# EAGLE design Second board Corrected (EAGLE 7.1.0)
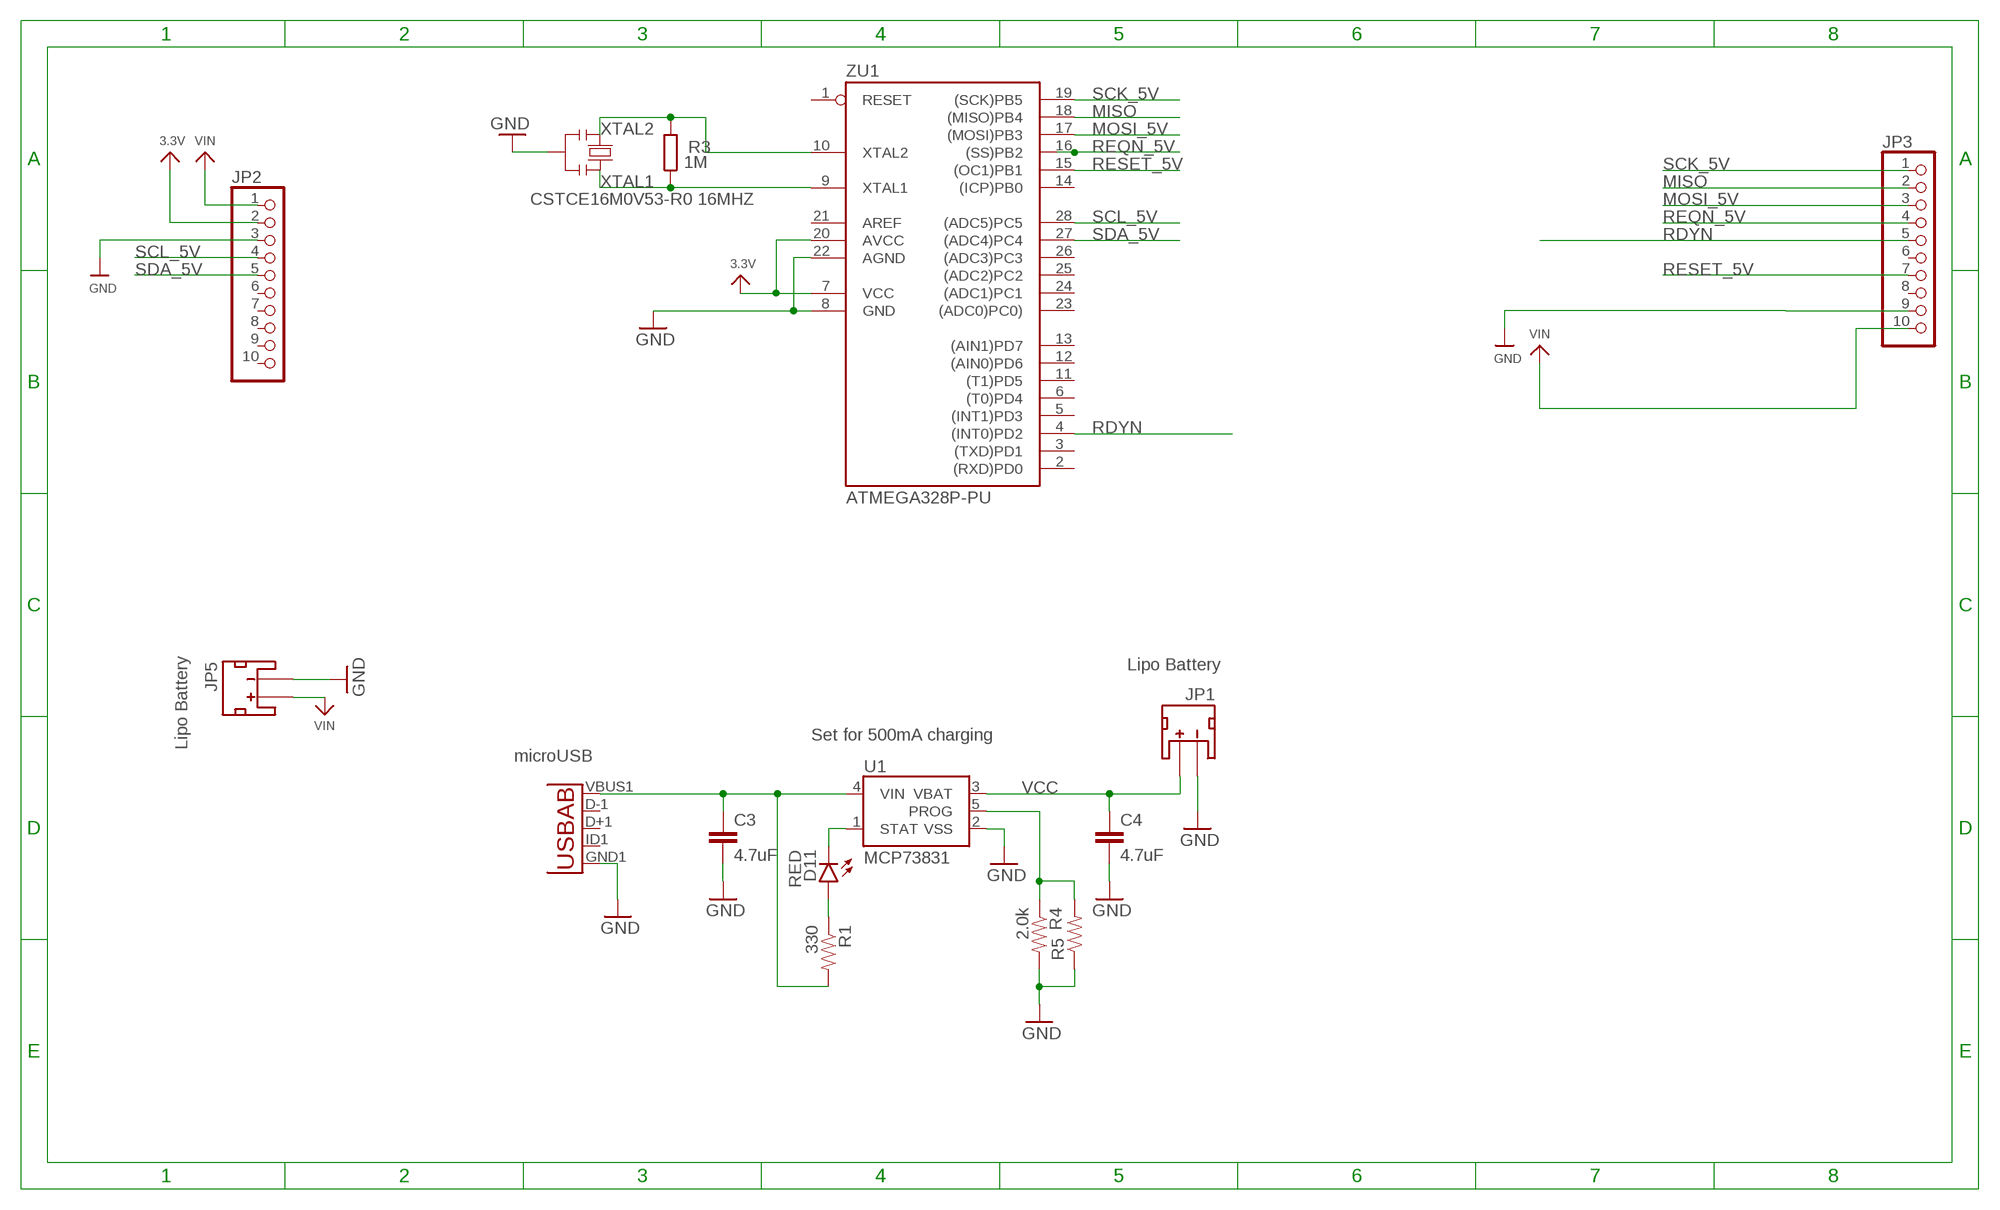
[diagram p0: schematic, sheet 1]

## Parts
C3  4.7uF  4.7UF-6.3V-10%(0603)0603  [0603-CAP]
C4  4.7uF  4.7UF-6.3V-10%(0603)0603  [0603-CAP]
D11  RED  LED-RED0603  [LED-0603]
JP1  JST  JST_2MM_MALE  [JST-2-SMD]
JP2  HEADER-1X10ROUND  [1X10_ROUND]
JP3  HEADER-1X1070MIL  [1X10_ROUND70]
JP5  JST  JST_2MM_MALE  [JST-2-SMD]
JP9  Micro USB  USB-ABCONN-11794  [USB-AB-MICRO-SMD_V03]
R1  330  330OHM1/10W1%(0603)  [0603-RES]
R3  1M  R-EU_R0603  [R0603-ROUND]
R4  2.0k  2.0KOHM1/10W5%(0603)  [0603-RES]
R5  RESISTORPTH-1/4W-VERT-KIT  [AXIAL-0.1EZ]
U1  MCP73831  [SOT23-5]
Y2  CSTCE16M0V53-R0 16MHZ  RESONATORMU  [RESONATOR]
ZU1  ATMEGA328P-PU  [DIL28-3]

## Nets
3.3V: JP2.2 ZU1.7(VCC) ZU1.20(AVCC)
GND: C3.2 C4.2 JP1.1(-) JP2.3 JP3.9 JP5.1(-) JP9.GND1(GND) R4.2 R5.P$1 U1.2(VSS) Y2.2 ZU1.8(GND) ZU1.22(AGND)
MISO: JP3.2 ZU1.18((MISO)PB4)
MOSI_5V: JP3.3 ZU1.17((MOSI)PB3)
N$3: D11.A R1.1
PROG: R4.1 R5.P$2 U1.5(PROG)
RDYN: JP3.5 ZU1.4((INT0)PD2)
REQN_5V: JP3.4 ZU1.16((SS)PB2)
RESET_5V: JP3.7 ZU1.15((OC1)PB1)
SCK_5V: JP3.1 ZU1.19((SCK)PB5)
SCL_5V: JP2.4 ZU1.28((ADC5)PC5)
SDA_5V: JP2.5 ZU1.27((ADC4)PC4)
STAT: D11.C U1.1(STAT)
USB: C3.1 JP9.VBUS1(VBUS) R1.2 U1.4(VIN)
VCC: C4.1 JP1.2(+) U1.3(VBAT)
VIN: JP2.1 JP3.10 JP5.2(+)
XTAL1: R3.1 Y2.3 ZU1.9(XTAL1)
XTAL2: R3.2 Y2.1 ZU1.10(XTAL2)
Unconnected: JP1.NC1(PAD1) JP1.NC2(PAD2) JP2.6 JP2.7 JP2.8 JP2.9 JP2.10 JP3.6 JP3.8 JP5.NC1(PAD1) JP5.NC2(PAD2) JP9.D+1(D+) JP9.D-1(D-) JP9.ID1(USBID) ZU1.1(RESET) ZU1.2((RXD)PD0) ZU1.3((TXD)PD1) ZU1.5((INT1)PD3) ZU1.6((T0)PD4) ZU1.11((T1)PD5) ZU1.12((AIN0)PD6) ZU1.13((AIN1)PD7) ZU1.14((ICP)PB0) ZU1.21(AREF) ZU1.23((ADC0)PC0)) ZU1.24((ADC1)PC1) ZU1.25((ADC2)PC2) ZU1.26((ADC3)PC3)

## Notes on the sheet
- Lipo Battery
- Set for 500mA charging
- Lipo Battery
- microUSB

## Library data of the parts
C3 C4 = SparkFun-Capacitors:4.7UF-6.3V-10%(0603): CAP-08280; PROD_ID: CAP-08280
D11 = SparkFun-LED:LED-RED: Assorted Red LEDs; PROD_ID: DIO-00819
JP1 JP5 = SparkFun-Connectors:JST_2MM_MALE: Mates to single-cell LiPo batteries. CONN-08352; PROD_ID: CONN-08352
JP2 JP3 = microbuilder:HEADER-1X10: PIN HEADER
JP9 = SparkFun-Connectors:USB-AB: This is a USB AB connector that is compatible with USB OTG. i.e. this connector can serve as a host or device; PROD_ID: CONN-11794
R1 = SparkFun-Resistors:330OHM1/10W1%(0603): RES-00818; PROD_ID: RES-00818
R3 = SmartPrj:R-EU_: RESISTOR, European symbol
R4 = SparkFun-Resistors:2.0KOHM1/10W5%(0603): RES-08296; PROD_ID: RES-08296
R5 = SparkFun-Resistors:RESISTOR: Resistor
U1 = SparkFun-PowerIC:MCP73831: Miniature single cell, fully integrated Li-Ion, Li-polymer charge management controller http://ww1.microchip.com/downloads/en/DeviceDoc/21984a.pdf IC-09995; PROD_ID: IC-09995
Y2 = SmartPrj:RESONATOR
ZU1 = SmartPrj:ATMEGA328P-: MICROCONTROLLER 4 Kbytes FLASH 128 bytes SRAM 256 bytes EEPROM UART 6-channel 10 bit ADC

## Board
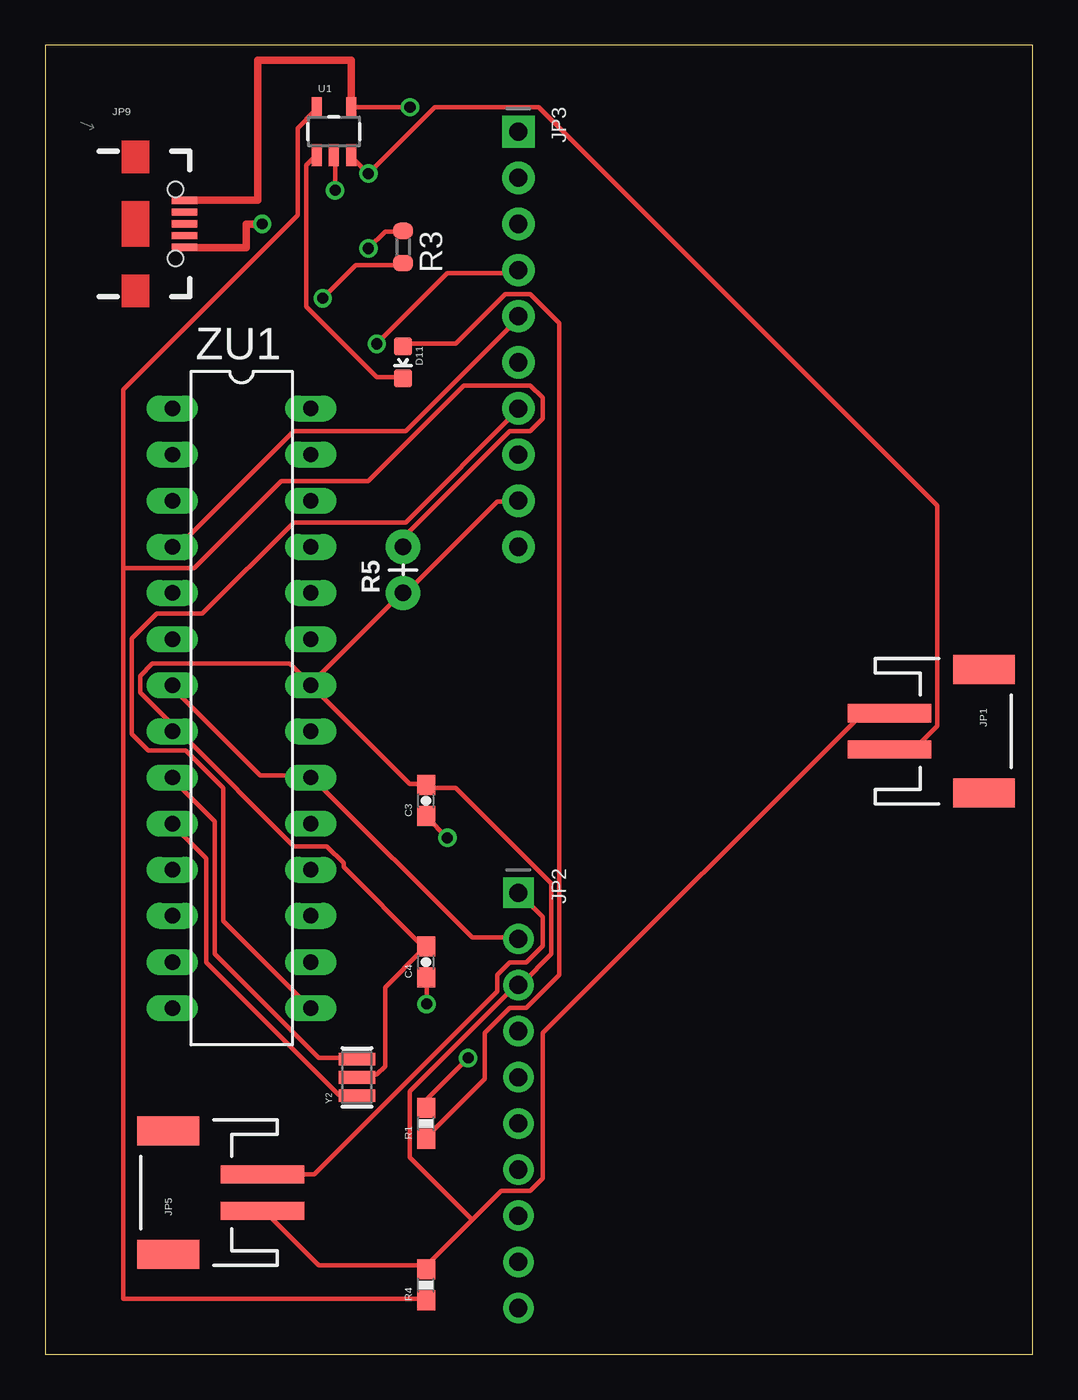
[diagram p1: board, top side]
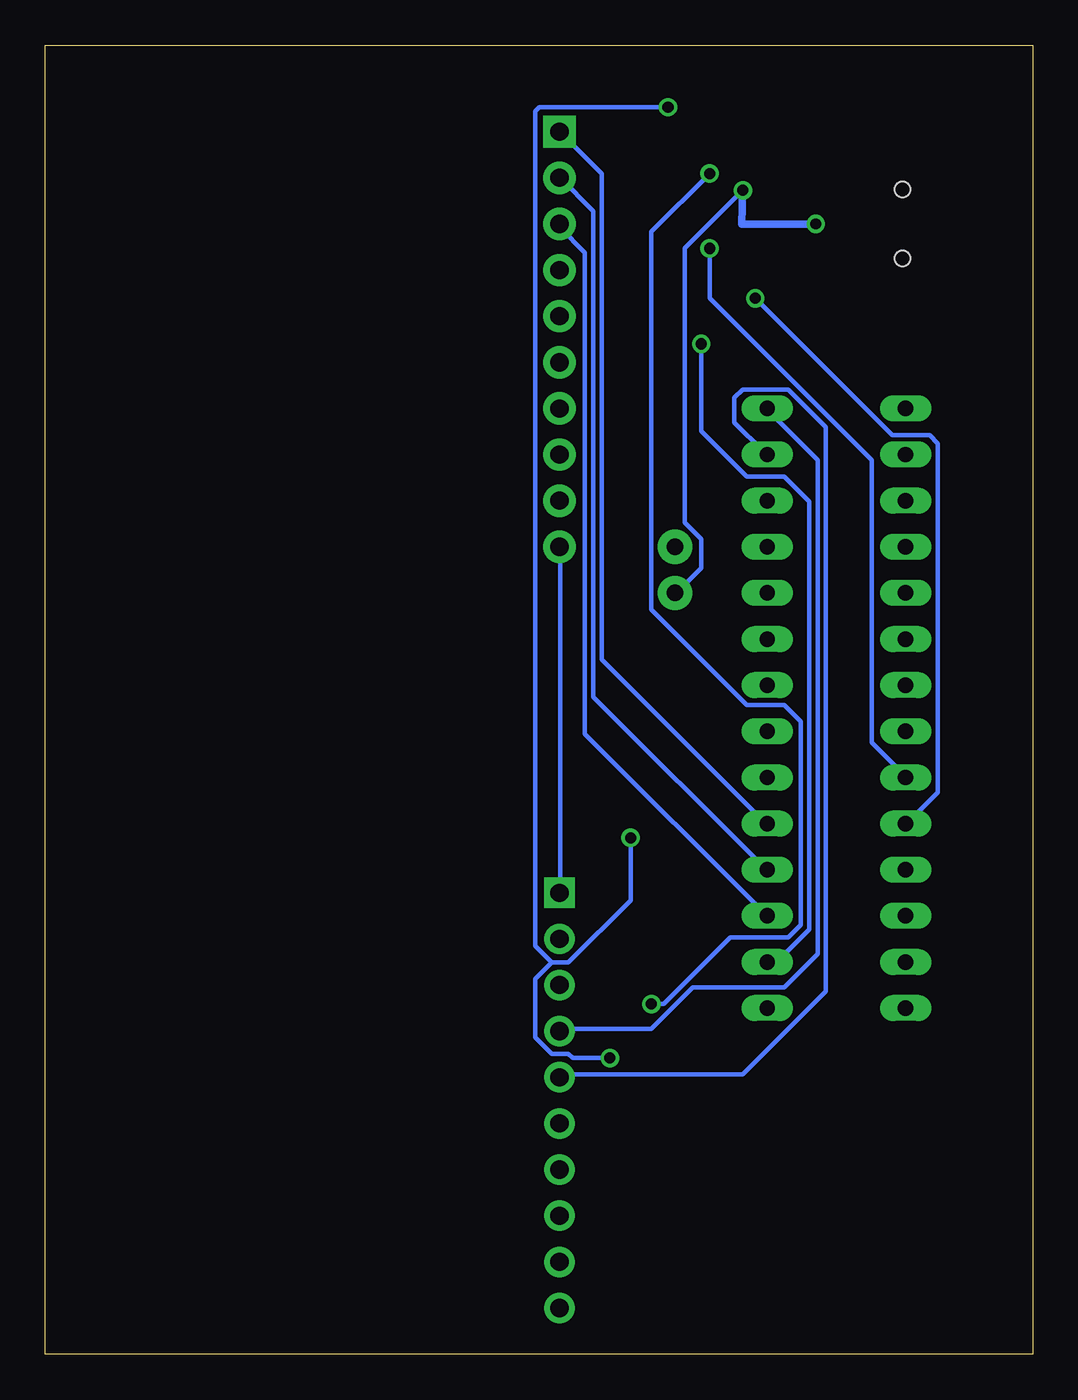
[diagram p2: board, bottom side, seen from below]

Size 54.34 x 72.06 mm. Coordinates in mm from the lower left corner, seen from the top.
Outline: 0,0 54.34,0 54.34,72.06 0,72.06 0,0
Copper layers (1*16): Top 0.035mm / dielectric 1.5mm / Bottom 0.035mm
Design rules "default": minimum track width 10mil, minimum drill 24mil, track to track 8mil, track to pad 8mil, pad to pad 8mil, via to via 8mil, smd to smd 8mil, copper to edge 40mil, drill to drill 8mil, minimum pad ring 10mil, minimum via ring 8mil, stop-mask expansion 4mil, vias tented up to drill 0mil, thermal gap 10mil

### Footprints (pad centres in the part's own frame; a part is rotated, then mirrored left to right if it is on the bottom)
0603-CAP = smd 1.1 x 1: 1 -0.85,0; 2 0.85,0
LED-0603 = smd 1 x 1: A 0,-0.877; C 0,0.877
JST-2-SMD = smd 1 x 4.6: 1 -1,-3.7; 2 1,-3.7 | smd 1.6 x 3.4: NC1 -3.4,1.5; NC2 3.4,1.5
1X10_ROUND = drill 1 pad 1.676 square: 1 -11.43,0 | drill 1 pad 1.676: 2 -8.89,0; 3 -6.35,0; 4 -3.81,0; 5 -1.27,0; 6 1.27,0; 7 3.81,0; 8 6.35,0; 9 8.89,0; 10 11.43,0
1X10_ROUND70 = drill 1 pad 1.778 square: 1 -11.43,0 | drill 1 pad 1.778: 2 -8.89,0; 3 -6.35,0; 4 -3.81,0; 5 -1.27,0; 6 1.27,0; 7 3.81,0; 8 6.35,0; 9 8.89,0; 10 11.43,0
USB-AB-MICRO-SMD_V03 = smd 1.4 x 0.4: D+1 2.7,0; D-1 2.7,0.65; GND1 2.7,-1.3; ID1 2.7,-0.65; VBUS1 2.7,1.3 | hole 0.85: 2.2,1.9; 2.2,-1.9
0603-RES = smd 1.1 x 1: 1 -0.85,0; 2 0.85,0
R0603-ROUND = smd 0.898 x 1.1: 1 -0.889,0; 2 0.889,0
AXIAL-0.1EZ = drill 0.9 pad 1.88: P$1 0,0; P$2 2.54,0
SOT23-5 = smd 0.55 x 1.2: 1 -0.95,-1.3; 2 0,-1.3; 3 0.95,-1.3; 4 0.95,1.3; 5 -0.95,1.3
RESONATOR = smd 0.7 x 2: 1 -1,0; 2 0,0; 3 1,0
DIL28-3 = drill 0.85 pad 1.422 long: 1 -16.51,-3.81; 2 -13.97,-3.81; 3 -11.43,-3.81; 4 -8.89,-3.81; 5 -6.35,-3.81; 6 -3.81,-3.81; 7 -1.27,-3.81; 8 1.27,-3.81; 9 3.81,-3.81; 10 6.35,-3.81; 11 8.89,-3.81; 12 11.43,-3.81; 13 13.97,-3.81; 14 16.51,-3.81; 15 16.51,3.81; 16 13.97,3.81; 17 11.43,3.81; 18 8.89,3.81; 19 6.35,3.81; 20 3.81,3.81; 21 1.27,3.81; 22 -1.27,3.81; 23 -3.81,3.81; 24 -6.35,3.81; 25 -8.89,3.81; 26 -11.43,3.81; 27 -13.97,3.81; 28 -16.51,3.81

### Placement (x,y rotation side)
C3  20.96,30.48 90 top
C4  20.96,21.59 90 top
D11  19.69,54.61 180 top
JP1  50.16,34.29 270 top
JP2  26.04,13.97 270 top
JP3  26.04,55.88 270 top
JP5  8.26,8.89 90 top
JP9  4.95,62.23 0 top
R1  20.96,12.7 90 top
R3  19.69,60.96 270 top
R4  20.96,3.81 90 top
R5  19.69,41.91 90 top
U1  15.88,67.31 0 top
Y2  17.15,15.24 90 top
ZU1  10.79,35.56 270 top

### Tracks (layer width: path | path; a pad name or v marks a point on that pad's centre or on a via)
3.3V
  Top 0.254: ZU1.7 7.04,36.65 11.84,31.85 14.58,31.85 ZU1.20 14.81,31.62 23.5,22.94 26.01,22.94 JP2.2
GND  (via drill 0.6, 0.61)
  Top 0.254: JP5.1 12.06,7.85 15.04,4.88 20.75,4.88 R4.2 20.98,4.88 23.5,7.39 | 23.5,7.39 25.1,8.99 26.7,8.99 27.38,9.68 27.38,17.68 44.98,35.28 46.35,35.28 JP1.1 | v15.95,64.08 15.95,65.91 U1.2 | JP3.9 26.01,46.94 24.87,46.94 19.84,41.91 R5.P$1 19.61,41.91 14.58,36.88 | Y2.2 17.32,15.39 18.24,15.39 18.69,15.85 18.69,20.19 20.75,22.25 C4.2 20.75,22.48 16.41,26.82 16.41,27.05 15.49,27.96 13.66,27.96 7.49,34.14 7.04,34.14 ZU1.8 6.81,34.37 6.81,34.82 5.21,36.42 5.21,37.34 5.89,38.02 13.44,38.02 14.58,36.88 | 14.58,36.88 ZU1.22 14.81,36.65 20.07,31.39 20.75,31.39 C3.2 20.98,31.17 22.58,31.17 27.84,25.91 27.84,22.02 26.24,20.42 JP2.3 26.01,20.42 20.07,14.48 20.07,10.82 23.5,7.39
  Top 0.406: JP9.GND1 11.05,60.93 11.05,62.23 v11.94,62.23
  Bottom 0.254: v15.95,64.08 19.15,60.88 19.15,45.8 18.24,44.88 18.24,43.28 19.61,41.91 R5.P$1
  Bottom 0.406: v11.94,62.23 16,62.23 v15.95,64.08
MISO
  Bottom 0.254: ZU1.18 14.81,26.82 24.18,36.2 24.18,62.94 26.01,64.77 JP3.2
MOSI_5V
  Bottom 0.254: ZU1.17 14.81,24.31 24.64,34.14 24.64,60.66 26.01,62.03 JP3.3
N$1  (via drill 0.6)
  other vias: 11.94,62.23
N$3
  Top 0.254: D11.A 19.84,55.63 22.58,55.63 25.32,58.37 26.7,58.37 28.3,56.77 28.3,20.88 26.47,19.05 25.55,19.05 24.18,17.68 24.18,15.16 20.98,11.96 R1.1
PROG
  Top 0.254: 4.29,43.28 4.29,53.11 13.89,62.71 13.89,67.51 14.81,68.43 U1.5 | 4.29,43.28 4.29,3.05 20.75,3.05 R4.1 | 4.29,43.28 8.18,43.28 12.98,48.08 17.78,48.08 23.04,53.34 26.7,53.34 27.38,52.65 27.38,51.51 26.7,50.83 25.55,50.83 19.84,45.11 19.84,44.65 R5.P$2
RDYN
  Top 0.254: ZU1.4 7.04,44.65 7.49,44.65 13.66,50.83 19.84,50.83 26.01,57 JP3.5
REQN_5V  (via drill 0.61)
  Top 0.254: v18.24,55.63 22.12,59.51 26.01,59.51 JP3.4
  Bottom 0.254: v18.24,55.63 18.24,50.83 15.72,48.31 13.66,48.31 12.29,46.94 12.29,23.39 13.89,21.79 14.58,21.79 ZU1.16
RESET_5V
  Top 0.254: ZU1.15 14.58,19.05 9.78,23.85 9.78,31.17 7.72,33.22 5.66,33.22 4.75,34.14 4.75,39.39 6.12,40.77 8.64,40.77 13.66,45.8 19.84,45.8 26.01,51.97 JP3.7
SCK_5V
  Bottom 0.254: JP3.1 23.72,65 23.72,38.25 14.81,29.34 ZU1.19
SCL_5V
  Bottom 0.254: ZU1.28 14.58,51.97 11.84,49.22 11.84,22.02 13.66,20.19 18.69,20.19 20.98,17.91 26.01,17.91 JP2.4
SDA_5V
  Bottom 0.254: ZU1.27 14.81,49.68 16.41,51.28 16.41,52.65 15.95,53.11 13.44,53.11 11.38,51.05 11.38,19.96 15.95,15.39 26.01,15.39 JP2.5
STAT
  Top 0.254: D11.C 19.61,53.8 18.24,53.8 14.35,57.68 14.35,65.46 14.81,65.91 U1.1
USB  (via drill 0.61)
  Top 0.254: v23.27,16.31 20.98,14.02 20.98,13.56 R1.2 | v22.12,28.42 20.98,29.57 C3.1 | v20.07,68.66 16.87,68.66 U1.4
  Top 0.406: JP9.VBUS1 11.68,63.53 11.68,71.25 16.83,71.25 U1.4
  Bottom 0.254: v23.27,16.31 25.32,16.31 25.55,16.53 26.47,16.53 27.38,17.45 27.38,20.65 26.47,21.56 | 26.47,21.56 25.55,21.56 22.12,24.99 v22.12,28.42 | v20.07,68.66 27.15,68.66 27.38,68.43 27.38,22.48 26.47,21.56
VCC  (via drill 0.61)
  Top 0.254: v20.98,19.28 20.98,20.65 C4.1 | U1.3 16.87,65.91 v17.78,65 21.44,68.66 27.15,68.66 49.1,46.71 49.1,34.59 47.95,33.45 46.58,33.45 JP1.2
  Bottom 0.254: v20.98,19.28 20.3,19.28 16.64,22.94 13.44,22.94 12.75,23.62 12.75,34.82 13.66,35.74 15.72,35.74 20.98,41 20.98,61.8 v17.78,65
VIN
  Top 0.254: JP5.2 12.06,9.91 14.81,9.91 24.87,19.96 24.87,20.88 25.55,21.56 26.47,21.56 27.38,22.48 27.38,24.08 26.24,25.22 JP2.1
  Bottom 0.254: JP2.1 26.01,25.45 26.01,44.42 JP3.10
XTAL1  (via drill 0.61)
  Top 0.254: v17.78,60.88 18.69,61.8 19.61,61.8 R3.1 | Y2.3 17.09,16.31 15.04,16.31 9.32,22.02 9.32,29.34 7.04,31.62 ZU1.9
  Bottom 0.254: v17.78,60.88 17.78,58.14 8.87,49.22 8.87,33.68 7.04,31.85 ZU1.9
XTAL2  (via drill 0.61)
  Top 0.254: v15.27,58.14 17.09,59.97 19.61,59.97 R3.2 | Y2.1 17.09,14.25 16.18,14.25 8.87,21.56 8.87,27.28 7.04,29.11 ZU1.10
  Bottom 0.254: v15.27,58.14 7.72,50.6 5.66,50.6 5.21,50.14 5.21,30.94 6.81,29.34 ZU1.10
